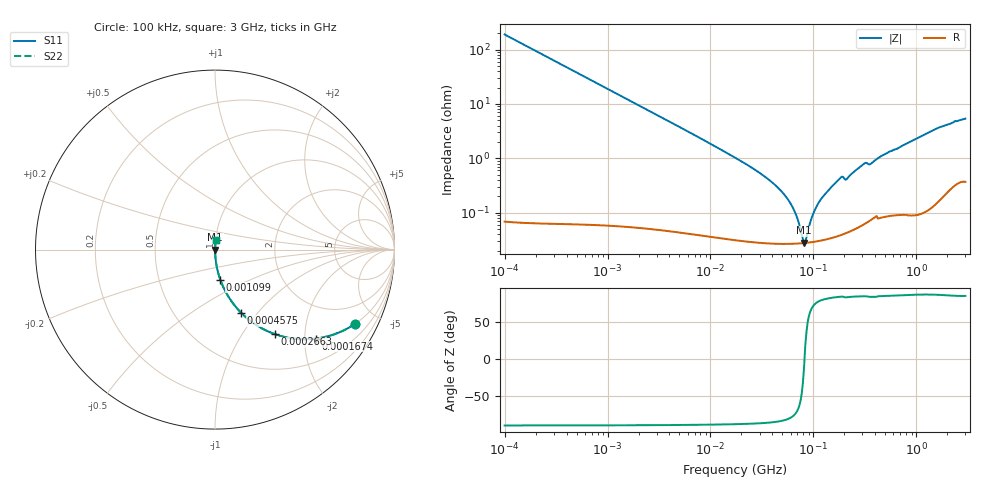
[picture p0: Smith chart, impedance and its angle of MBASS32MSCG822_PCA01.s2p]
! MBASS32MSCG822_PCA01  S-PARAMETER MODEL  ( Standard Model )
! Model Generated by TAIYO YUDEN Corporation (https://www.yuden.co.jp/en/)
! Version 1.0
! TAIYO YUDEN Control No. 250312
! Copyright(c) 2025 TAIYO YUDEN CO.,LTD. All Rights Reserved.
! Product Description (link to TY-COMPAS)
! https://ds.yuden.co.jp/TYCOMPAS/or/detail?pn=MBASS32MSCG822JPCA01&u=M
! Products Name : Multilayer Ceramic Capacitors
! Characteristics :
!  Capacitance : 8200 [pF] , Rated Voltage : 630 [V] , TCC : CG / C0G
!  Case Size : 3.2 x 2.5 / 0.126 x 0.098 [mm/inch] , Thickness : 2.5 / 0.098 [mm/inch]
!  (Conditions: Temperature = 25 [degC] , DC Bias Voltage = 0 [V])
! External Node Assignments :
!  1  o---| |---o  2
! GND o---------o GND
! Frequency Range : 0.1MHz  -  3000MHz  [ 401 STEP ]
# MHZ S RI R 50
! Freq[MHz].  S11 Real  S11 Imag  S21 Real  S21 Imag  S12 Real  S12 Imag  S22 Real  S22 Imag
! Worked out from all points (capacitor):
!   401 points, 100 kHz to 3 GHz, reference 50 ohm
!   read as one part in series: C = 8.41 nF near 105.3 kHz
!   lowest |Z| = 28 mohm at 81.31 MHz (marker M1)
!   series resonance near 82.02 MHz, so ESL is about 450 pH
!   S11 on the Smith chart (normalised r, x): 100 kHz: 1.00, -3.79; 167.4 kHz: 1.00, -2.26; 266.3 kHz: 1.00, -1.42; 457.5 kHz: 1.00, -0.83; 1.099 MHz: 1.00, -0.34; 3 GHz: 1.01, +0.11
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0.1  0.7821 -0.4127  0.2179 0.4127  0.2179 0.4127  0.7821 -0.4127
0.167439  0.5612 -0.496  0.4388 0.496  0.4388 0.496  0.5612 -0.496
0.266273  0.336 -0.4719  0.664 0.4719  0.664 0.4719  0.336 -0.4719
0.457483  0.1466 -0.3529  0.8534 0.3529  0.8534 0.3529  0.1466 -0.3529
0.562235  0.1023 -0.3022  0.8977 0.3022  0.8977 0.3022  0.1023 -0.3022
1.09883  0.0294 -0.1672  0.9706 0.1672  0.9706 0.1672  0.0294 -0.1672
3.161081  0.00404 -0.0595  0.996 0.0595  0.996 0.0595  0.00404 -0.0595
17.7727  0.000409 -0.00999  0.9996 0.00999  0.9996 0.00999  0.000409 -0.00999
33.85116  0.000294 -0.00457  0.9997 0.00457  0.9997 0.00457  0.000294 -0.00457
51.12795  0.000271 -0.00223  0.9997 0.00223  0.9997 0.00223  0.000271 -0.00223
64.47533  0.000269 -0.00111  0.9997 0.00111  0.9997 0.00111  0.000269 -0.00111
81.30716  0.000276 -4.7e-05  0.9997 4.7e-05  0.9997 4.7e-05  0.000276 -4.7e-05
85.60801  0.000279 0.000205  0.9997 -0.000205  0.9997 -0.000205  0.000279 0.000205
97.38194  0.000288 0.000802  0.9997 -0.000802  0.9997 -0.000802  0.000288 0.000802
119.6798  0.00031 0.00179  0.9997 -0.00179  0.9997 -0.00179  0.00031 0.00179
180.7614  0.000398 0.00423  0.9996 -0.00423  0.9996 -0.00423  0.000398 0.00423
210.9903  0.000441 0.00413  0.9996 -0.00413  0.9996 -0.00413  0.000441 0.00413
310.5665  0.000672 0.0079  0.9993 -0.0079  0.9993 -0.0079  0.000672 0.0079
362.5028  0.000794 0.00789  0.9992 -0.00789  0.9992 -0.00789  0.000794 0.00789
547.5153  0.00104 0.0132  0.999 -0.0132  0.999 -0.0132  0.00104 0.0132
1575.075  0.0027 0.035  0.9973 -0.035  0.9973 -0.035  0.0027 0.035
3000  0.0065 0.053  0.9935 -0.053  0.9935 -0.053  0.0065 0.053
